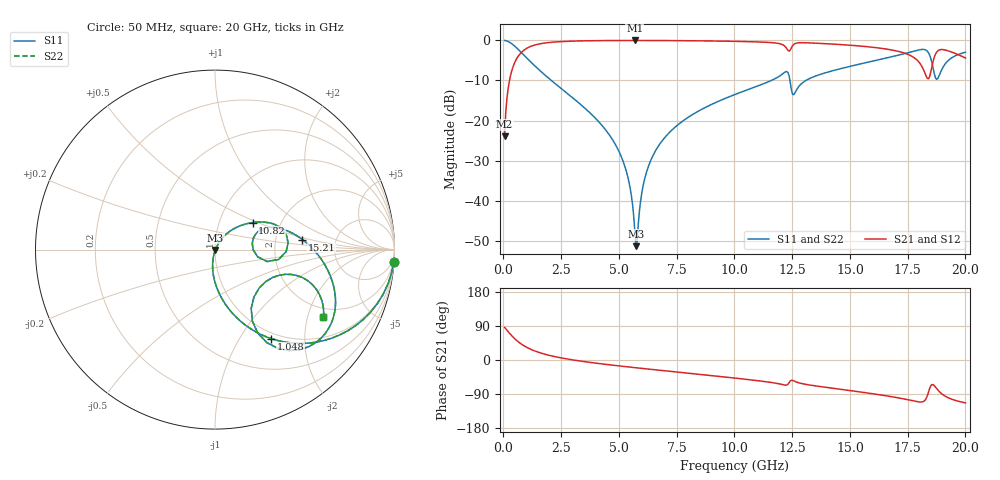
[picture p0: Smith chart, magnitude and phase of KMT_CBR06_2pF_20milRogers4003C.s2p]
! Data measured by Modelithics Inc. support@modelithics.com 813-866-6335
! KEMET CBR0603 2pF, Pad Width= 0.851mm, Pad Length= 0.64mm, Pad Gap= 0.62mm, 20mil Rogers 4003C substrate Data, January 2022
# hz S ma R 50
! 2 Port Network Data from SP1.SP block
! freq  magS11  angS11  magS21  angS21  magS12  angS12  magS22  angS22
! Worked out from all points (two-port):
!   401 points, 50 MHz to 20 GHz, reference 50 ohm
!   highest |S21| = -0.02 dB at 5.686 GHz (marker M1); lowest = -23.9 dB at 50 MHz (marker M2)
!   |S21| within 3 dB of the highest: 772.7 MHz to 17.28 GHz (16.51 GHz wide, 183 % of centre); 18.75 GHz to 19.46 GHz (712.7 MHz wide, 3.73 % of centre)
!   lowest |S11| = -51.3 dB at 5.736 GHz (marker M3), VSWR 1.01, Z = 50.2 - j0.173 ohm
!   |S11| at or under -10 dB: 2.074 GHz to 11.6 GHz (9.526 GHz wide, 139 % of centre); 12.4 GHz to 13.09 GHz (690.6 MHz wide, 5.42 % of centre)
!   |S22| runs from -51.3 to 0.0 dB; largest |S21 - S12| = 0
!   S11 on the Smith chart (normalised r, x): 50 MHz: 1, -30; 1.048 GHz: 0.91, -1.39; 10.82 GHz: 1.44, +0.46; 15.21 GHz: 2.85, +0.42; 20 GHz: 1.67, -2.52
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5e7  0.998 -3.8  0.06351 86.2  0.06351 86.2  0.998 -3.8
3.99125e8  0.8903 -28.5  0.4542 61.5  0.4542 61.5  0.8903 -28.5
1.0475e9  0.5877 -57.6  0.8077 32.2  0.8077 32.2  0.5877 -57.6
3.391625e9  0.1543 -92.5  0.9858 -3.3  0.9858 -3.3  0.1543 -92.5
5.0375e9  0.03917 -102.3  0.9966 -15.8  0.9966 -15.8  0.03917 -102.3
5.4365e9  0.01701 -100.0  0.9972 -18.5  0.9972 -18.5  0.01701 -100.0
5.685875e9  0.004334 -74.0  0.9972 -20.2  0.9972 -20.2  0.004334 -74.0
5.73575e9  0.002716 -39.4  0.9972 -20.5  0.9972 -20.5  0.002716 -39.4
6.13475e9  0.01979 59.2  0.9969 -23.1  0.9969 -23.1  0.01979 59.2
6.73325e9  0.04928 59.9  0.9958 -26.9  0.9958 -26.9  0.04928 59.9
1.0025e10  0.2117 41.2  0.973 -47.7  0.973 -47.7  0.2117 41.2
1.0823e10  0.258 35.7  0.9606 -53.2  0.9606 -53.2  0.258 35.7
1.22195e10  0.4066 10.5  0.8254 -66.3  0.8254 -66.3  0.4066 10.5
1.2419e10  0.2979 -12.9  0.7591 -55.2  0.7591 -55.2  0.2979 -12.9
1.336662e10  0.3458 21.1  0.927 -67.1  0.927 -67.1  0.3458 21.1
1.5212e10  0.4904 6.5  0.8613 -82.3  0.8613 -82.3  0.4904 6.5
1.670825e10  0.6154 -7.6  0.7687 -95.8  0.7687 -95.8  0.6154 -7.6
1.8005e10  0.7624 -30.6  0.5291 -110.8  0.5291 -110.8  0.7624 -30.6
1.835412e10  0.7316 -49.6  0.3352 -93.9  0.3352 -93.9  0.7316 -49.6
1.865338e10  0.385 -58.4  0.6175 -67.7  0.6175 -67.7  0.385 -58.4
1.90025e10  0.447 -18.1  0.7689 -90.5  0.7689 -90.5  0.447 -18.1
2e10  0.7111 -31.8  0.6028 -113.1  0.6028 -113.1  0.7111 -31.8
